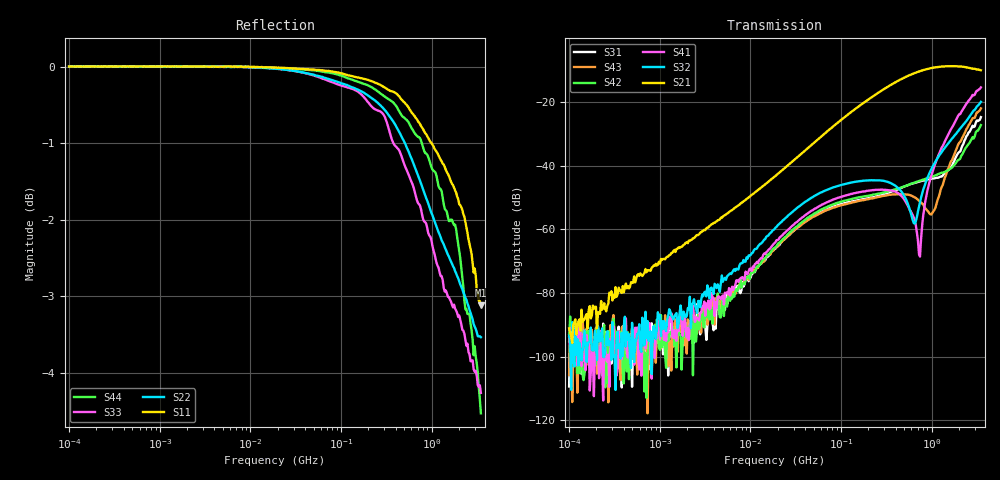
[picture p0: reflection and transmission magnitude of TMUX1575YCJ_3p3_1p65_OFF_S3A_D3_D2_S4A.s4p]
!Keysight Technologies,E5080A,MY55200740,A.12.60.03
!Date: Tuesday, July 21, 2020 11:54:04
!Correction: S11(Full 4 Port(1,2,3,4))
!S12(Full 4 Port(1,2,3,4))
!S13(Full 4 Port(1,2,3,4))
!S14(Full 4 Port(1,2,3,4))
!S21(Full 4 Port(1,2,3,4))
!S22(Full 4 Port(1,2,3,4))
!S23(Full 4 Port(1,2,3,4))
!S24(Full 4 Port(1,2,3,4))
!S31(Full 4 Port(1,2,3,4))
!S32(Full 4 Port(1,2,3,4))
!S33(Full 4 Port(1,2,3,4))
!S34(Full 4 Port(1,2,3,4))
!S41(Full 4 Port(1,2,3,4))
!S42(Full 4 Port(1,2,3,4))
!S43(Full 4 Port(1,2,3,4))
!S44(Full 4 Port(1,2,3,4))
!S4P File: Measurements: <S11,S12,S13,S14>,
!<S21,S22,S23,S24>,
!<S31,S32,S33,S34>,
!<S41,S42,S43,S44>:Log Frequency Sweep
# Hz S  dB  R 50
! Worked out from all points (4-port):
!   400 points, 100 kHz to 3.5 GHz, reference 50 ohm
!   strongest paths, dB at 100 kHz, 1.377 MHz, 18.96 MHz, 261 MHz, 3.5 GHz:
!     S21: -91.1, -67.4, -43.2, -17.0, -10.1
!     S32: -93.4, -87.6, -59.5, -44.6, -20.0
!     S41: -93.8, -93.5, -64.1, -47.6, -15.4
!     S42: -95.2, -90.4, -65.6, -48.8, -27.3
!     S43: -105.8, -93.1, -65.9, -49.8, -22.1
!     S31: -109.4, -96.5, -66.1, -49.5, -24.8
!   lowest |S11| = -3.1 dB at 3.5 GHz (marker M1), VSWR 5.64, Z = 11.8 - j28.2 ohm
!   |S11| at or under -10 dB: nowhere
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100000  0.00 -0.0  -89.56 139.3  -94.06 -77.6  -113.72 127.3
        -91.14 84.2  0.00 -0.0  -92.62 85.6  -93.16 -28.7
        -109.38 -30.5  -93.36 80.9  0.00 -0.0  -118.52 52.4
        -93.84 -1.8  -95.16 68.1  -105.85 -52.8  0.00 -0.0
4599829  -0.00 -0.4  -56.81 94.9  -84.17 96.8  -81.13 98.0
         -56.94 95.8  -0.01 -0.7  -77.42 108.6  -84.02 112.5
         -86.81 107.7  -79.68 106.9  0.00 -0.7  -82.44 114.6
         -81.32 114.5  -87.64 132.4  -82.72 123.5  -0.00 -0.4
2.229773e8  -0.20 -14.9  -18.33 77.5  -50.01 36.8  -47.72 38.3
            -18.33 77.5  -0.42 -24.5  -44.63 27.5  -49.21 34.1
            -50.02 36.7  -44.64 27.5  -0.53 -26.4  -50.34 35.1
            -47.71 38.4  -49.18 33.9  -50.33 34.9  -0.28 -16.7
4.896885e8  -0.46 -30.7  -12.50 54.2  -46.70 28.1  -50.35 25.7
            -12.50 54.2  -0.96 -49.0  -49.08 15.2  -46.64 25.2
            -46.68 28.2  -49.10 15.4  -1.25 -52.9  -48.99 19.2
            -50.33 26.0  -46.64 25.4  -49.04 19.3  -0.66 -34.7
7.44969e8  -0.75 -44.0  -10.34 38.4  -44.99 10.4  -68.42 143.5
           -10.34 38.3  -1.49 -66.8  -51.61 132.6  -44.74 13.2
           -44.96 10.5  -51.65 132.6  -1.81 -72.0  -51.29 -3.5
           -68.59 144.7  -44.77 13.5  -51.26 -3.5  -0.94 -48.3
1.103997e9  -1.09 -59.5  -9.14 22.3  -43.90 -26.9  -39.21 -171.7
            -9.14 22.4  -2.06 -84.4  -38.69 142.1  -43.09 -10.3
            -43.90 -27.1  -38.69 142.0  -2.50 -90.9  -53.06 -105.4
            -39.20 -171.6  -43.08 -10.4  -53.19 -105.0  -1.38 -63.9
3.5e9  -3.11 -119.1  -10.06 -19.2  -24.73 157.1  -15.43 128.7
       -10.06 -19.2  -3.53 -129.5  -19.94 136.2  -27.27 174.5
       -24.78 157.1  -19.99 136.3  -4.26 -140.6  -22.04 137.7
       -15.44 128.6  -27.28 174.3  -22.06 137.6  -4.52 -123.3
